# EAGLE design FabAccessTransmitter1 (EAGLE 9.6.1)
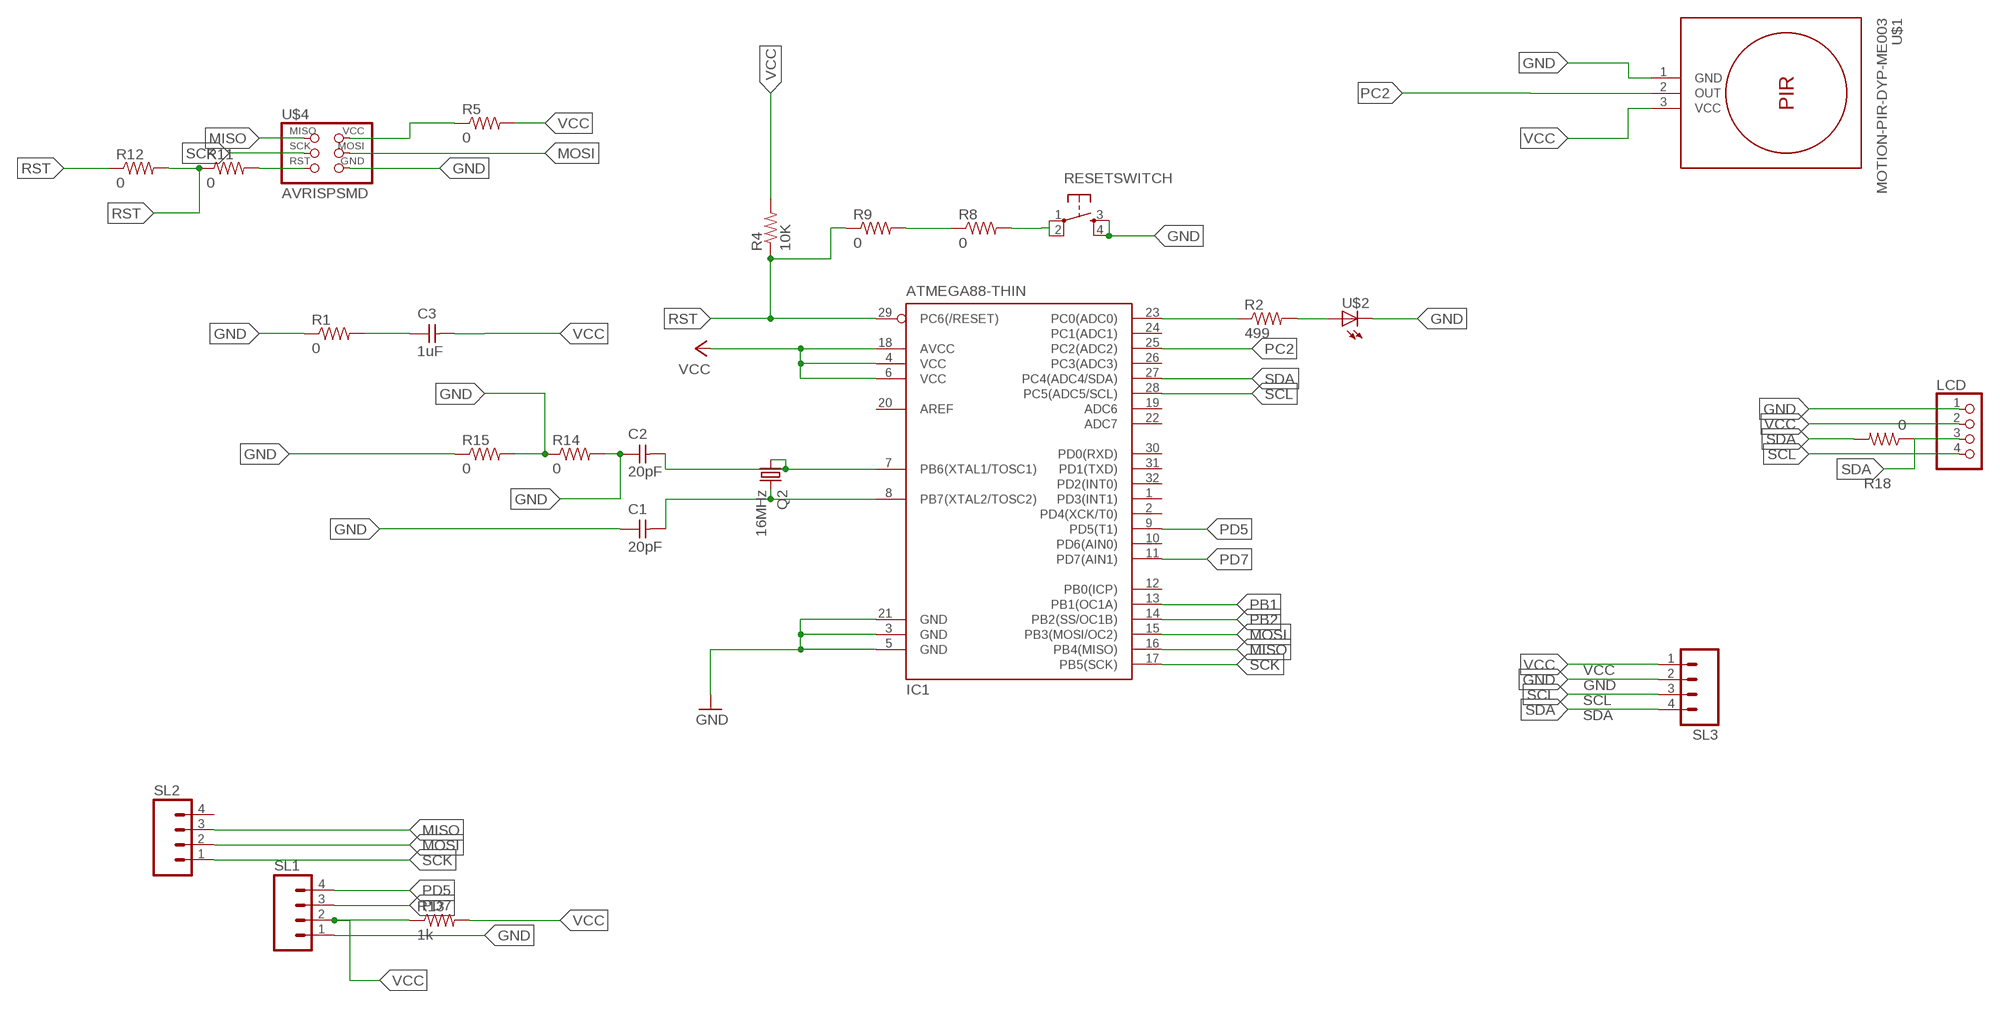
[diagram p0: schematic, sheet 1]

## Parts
C1  20pF  UNPOLARIZED_CAPACITOR1206  [1206]
C2  20pF  UNPOLARIZED_CAPACITOR1206  [1206]
C3  1uF  UNPOLARIZED_CAPACITOR1206  [1206]
IC1  ATMEGA88-THIN  [TQFP32-08THIN]
LCD  PINHD-1X4  [1X04]
Q2  16MHz  CSM-7X-DU  [CSM-7X-DU]
R1  0  RES-US1206  [R1206]
R2  499  RES-US1206  [R1206]
R4  10K  RESISTOR1206  [1206]
R5  0  RES-US1206  [R1206]
R8  0  RES-US1206  [R1206]
R9  0  RES-US1206  [R1206]
R11  0  RES-US1206  [R1206]
R12  0  RES-US1206  [R1206]
R13  1k  RES-US1206  [R1206]
R14  0  RES-US1206  [R1206]
R15  0  RES-US1206  [R1206]
R18  0  RESISTOR1206  [1206]
RESETSWITCH  6MM_SWITCH6MM_SWITCH  [6MM_SWITCH]
SL1  M04  [04P]
SL2  M04  [04P]
SL3  M04  [04P]
U$1  MOTION-PIR-DYP-ME003  [MOTION-PIR-DYP-ME003]
U$2  LED1206  [1206]
U$4  AVRISPSMD  [2X03SMD]

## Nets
GND: C1.1 C2.1 C3.1 IC1.3(GND) IC1.5(GND) IC1.21(GND) LCD.1 R1.1 R1.2 R14.1 R14.2 R15.1 R15.2 RESETSWITCH.3(S) RESETSWITCH.4(S1) SL1.1 SL3.2 U$1.1(GND) U$2.2(C) U$4.6(GND)
MISO: IC1.16(PB4(MISO)) SL2.3 U$4.1(MISO)
MOSI: IC1.15(PB3(MOSI/OC2)) SL2.2 U$4.4(MOSI)
N$1: IC1.23(PC0(ADC0)) R2.1
N$2: R2.2 U$2.1(A)
N$6: R8.1 R9.2
N$9: R8.2 RESETSWITCH.1(P) RESETSWITCH.2(P1)
PB1: IC1.13(PB1(OC1A))
PB2: IC1.14(PB2(SS/OC1B))
PC2: IC1.25(PC2(ADC2)) U$1.2(OUT)
PD5: IC1.9(PD5(T1)) SL1.4
PD7: IC1.11(PD7(AIN1)) SL1.3
RST: IC1.29(PC6(/RESET)) R4.1 R9.1 R11.1 R11.2 R12.1 R12.2 U$4.5(RST)
SCK: IC1.17(PB5(SCK)) SL2.1 U$4.3(SCK)
SCL: IC1.28(PC5(ADC5/SCL)) LCD.4 SL3.3
SDA: IC1.27(PC4(ADC4/SDA)) LCD.3 R18.1 R18.2 SL3.4
VCC: C3.2 IC1.4(VCC) IC1.6(VCC) IC1.18(AVCC) LCD.2 R4.2 R5.1 R5.2 R13.1 R13.2 SL1.2 SL3.1 U$1.3(VCC) U$4.2(VCC)
XTAL1: C2.2 IC1.7(PB6(XTAL1/TOSC1)) Q2.1
XTAL2: C1.2 IC1.8(PB7(XTAL2/TOSC2)) Q2.2
Unconnected: IC1.1(PD3(INT1)) IC1.2(PD4(XCK/T0)) IC1.10(PD6(AIN0)) IC1.12(PB0(ICP)) IC1.19(ADC6) IC1.20(AREF) IC1.22(ADC7) IC1.24(PC1(ADC1)) IC1.26(PC3(ADC3)) IC1.30(PD0(RXD)) IC1.31(PD1(TXD)) IC1.32(PD2(INT0)) SL2.4

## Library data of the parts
C1-C3 = FAB_Hello:UNPOLARIZED_CAPACITOR: unpolarized_capacitor
IC1 = fab:ATMEGA88-THIN
LCD = pinhead:PINHD-1X4: PIN HEADER
Q2 = FAB_Hello:CSM-7X-DU: SMD CRYSTAL; OC_FARNELL: unknown; OC_NEWARK: unknown
R1 R2 R5 R8 R9 R11-R15 = fab:RES-US: Resistor (US Symbol)
R4 R18 = FAB_Hello:RESISTOR
RESETSWITCH = FAB_Hello:6MM_SWITCH: OMRON SWITCH
SL1-SL3 = con-amp-quick:M04: AMP QUICK CONNECTOR; OC_FARNELL: unknown; OC_NEWARK: unknown
U$1 = diy-modules:MOTION-PIR-DYP-ME003: PIR Motion Sensor Module DYP-ME003 based on BISS0001 pyroelectic detector Click here to find device on ebay.com
U$2 = FAB_Hello:LED
U$4 = FAB_Hello:AVRISP

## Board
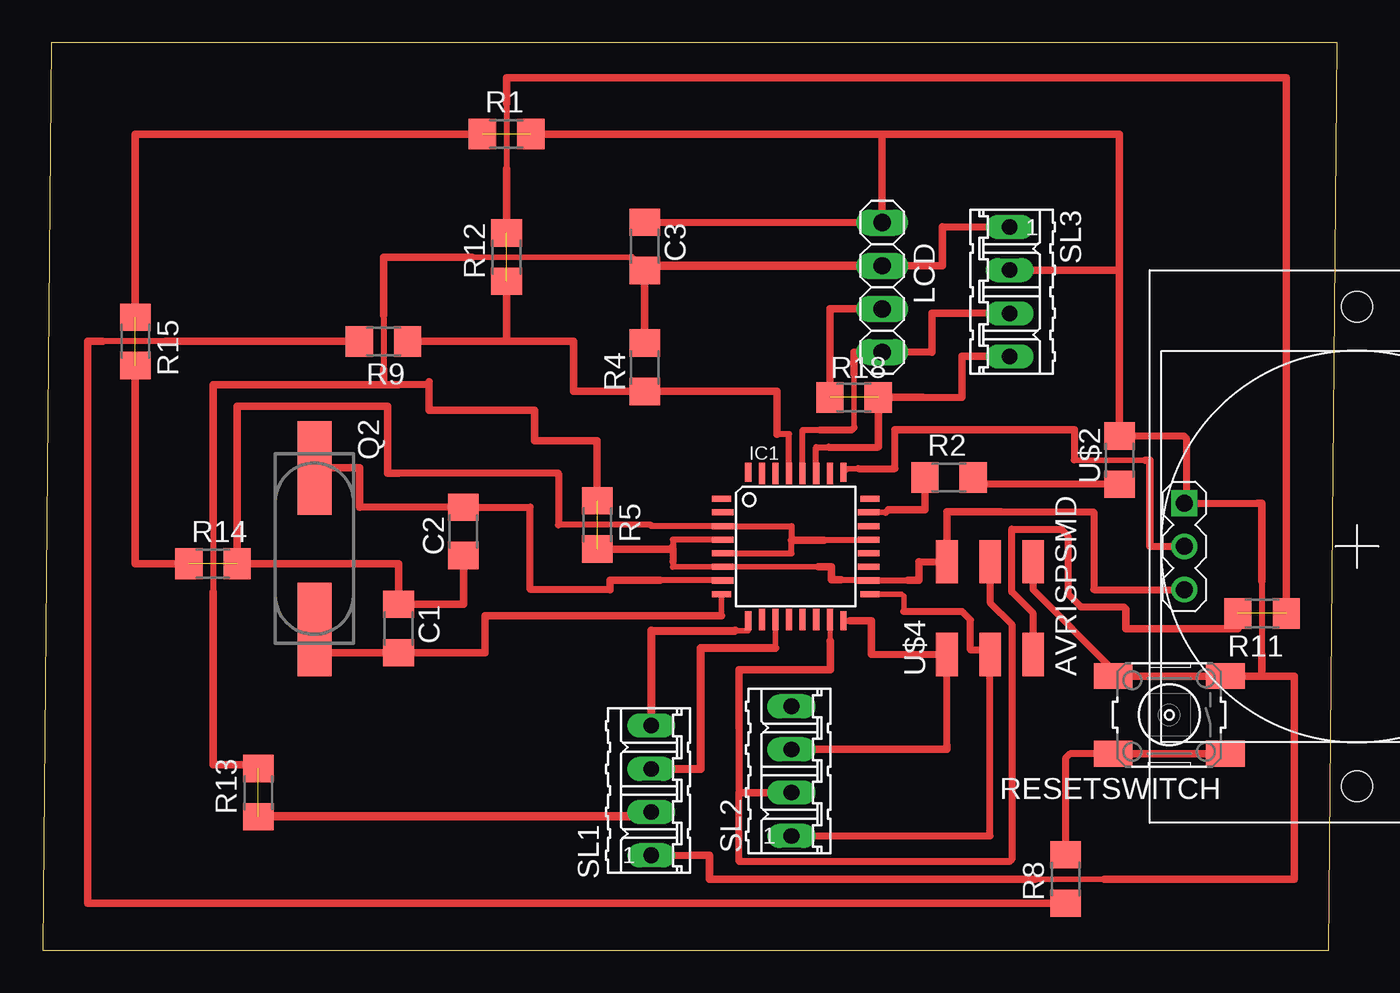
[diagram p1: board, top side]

Size 76.18 x 53.39 mm. Coordinates in mm from the lower left corner, seen from the top.
Outline: 0,0 75.67,0 76.18,53.39 0.51,53.39 0,0
Copper layers (1*16): Top 0.035mm / dielectric 1.5mm / Bottom 0.035mm
Design rules "default *": minimum track width 6mil, minimum drill 0.35mm, track to track 17mil, track to pad 17mil, pad to pad 17mil, via to via 17mil, smd to smd 17mil, copper to edge 40mil, drill to drill 6mil, minimum pad ring 10mil, minimum via ring 8mil, stop-mask expansion 4mil, vias tented up to drill 0mil, thermal gap 17mil

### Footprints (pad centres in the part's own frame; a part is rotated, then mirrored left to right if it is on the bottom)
1206 = smd 1.6 x 1.803: 1 -1.422,0; 2 1.422,0
TQFP32-08THIN = smd 1.118 x 0.356: 1 -4.369,2.8; 8 -4.369,-2.8; 17 4.369,-2.8; 24 4.369,2.8 | smd 1.27 x 0.356: 2 -4.293,2; 3 -4.293,1.2; 4 -4.293,0.4; 5 -4.293,-0.4; 6 -4.293,-1.2; 7 -4.293,-2; 18 4.293,-2; 19 4.293,-1.2; 20 4.293,-0.4; 21 4.293,0.4; 22 4.293,1.2; 23 4.293,2 | smd 0.356 x 1.118: 9 -2.8,-4.369; 16 2.8,-4.369; 25 2.8,4.369; 32 -2.8,4.369 | smd 0.356 x 1.27: 10 -2,-4.293; 14 1.2,-4.293; 15 2,-4.293; 26 2,4.293; 27 1.2,4.293; 31 -2,4.293 | smd 0.35 x 1.27: 11 -1.2,-4.293; 12 -0.4,-4.293; 13 0.4,-4.293; 28 0.4,4.293; 29 -0.4,4.293; 30 -1.2,4.293
1X04 = drill 1.016 long: 1 -3.81,0; 2 -1.27,0; 3 1.27,0; 4 3.81,0
CSM-7X-DU = smd 5.5 x 2: 1 -4.75,0; 2 4.75,0
R1206 = smd 1.6 x 1.803: 1 -1.422,0; 2 1.422,0
6MM_SWITCH = smd 2.286 x 1.524: 1 -3.302,2.286; 2 3.302,2.286; 3 -3.302,-2.286; 4 3.302,-2.286
04P = drill 0.914 long: 1 -3.81,0; 2 -1.27,0; 3 1.27,0; 4 3.81,0
MOTION-PIR-DYP-ME003 = drill 1 square: 1 -2.54,-10.16 | drill 1: 2 0,-10.16; 3 2.54,-10.16 | hole 1.8: -14.1,0; 14.1,0
2X03SMD = smd 2.54 x 1.27: 1 -2.54,2.54; 2 2.92,2.54; 3 -2.54,0; 4 2.92,0; 5 -2.54,-2.54; 6 2.92,-2.54

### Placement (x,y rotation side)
C1  20.96,18.92 270 top
C2  24.77,24.64 90 top
C3  35.43,41.4 270 top
IC1  44.32,23.75 0 top
LCD  49.4,38.99 270 top
Q2  16,23.62 270 top
R1  27.31,48.01 0 top
R2  53.34,27.81 0 top
R4  35.43,34.29 90 top
R5  32.64,25.02 270 top
R8  60.2,4.19 90 top
R9  20.07,35.81 180 top
R11  71.75,19.81 180 top
R12  27.31,40.77 90 top
R13  12.7,9.27 90 top
R14  10.03,22.73 0 top
R15  5.46,35.81 270 top
R18  47.75,32.51 0 top
RESETSWITCH  66.29,13.84 180 top
SL1  35.81,9.4 90 top
SL2  44.07,10.54 90 top
SL3  56.9,38.73 270 top
U$1  77.34,23.75 270 top
U$2  63.37,28.83 90 top
U$4  55.75,19.94 90 top

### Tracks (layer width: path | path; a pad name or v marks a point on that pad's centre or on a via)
GND  (3 unrouted)
  Top 0.33: 58.42,4.19 62.48,4.19 64.13,4.19 | IC1.21 48.62,24.13 47.75,24.13
  Top 0.356: 30.35,25.02 35.81,25.02 35.81,24.95 IC1.3 44.07,24.95 44.07,24.13 44.07,23.35 IC1.5 | 47.75,24.13 45.97,24.13 | 71.75,25.4 71.75,21.72 71.75,17.4
  Top 0.406: U$4.6 58.29,21.21 62.99,16.51 RESETSWITCH.4 64.01,16.13 | 67.31,26.29 71.5,26.29 | 67.31,26.29 U$1.1 | LCD.1 35.45,42.8 C3.1 | SL1.1 38.23,5.59 | 63.37,31.62 U$2.2 67.16,30.25 67.31,30.1 67.31,26.29 | 30.35,25.02 30.35,28.07 20.96,28.07 | R14.1 8.13,23.22
  Top 0.432: 71.75,17.4 71.75,16.13 | 45.97,24.13 44.07,24.13 | R14.1 5.46,22.73 R15.2 | C2.1 24.77,20.35 C1.1 20.96,22.73 R14.2 11.46,32 20.32,32 20.32,28.07 20.96,28.07 | R1.2 49.4,48.01 | 49.4,48.01 LCD.1 | 49.4,48.01 63.37,48.01 63.37,40 | 63.37,40 U$2.2 | SL3.2 63.37,40 | R1.1 5.46,48.01 R15.1 | 38.23,5.59 39.24,5.59 39.24,4.19 58.42,4.19 | 71.5,26.29 71.75,26.29 71.75,21.72 | RESETSWITCH.4 RESETSWITCH.3 71.75,16.13 | 62.48,4.19 73.66,4.19 73.66,16.13 71.75,16.13
MISO
  Top 0.356: IC1.16 47.5,19.38
  Top 0.406: 53.21,12.07 U$4.1 48.77,17.4
  Top 0.432: 47.5,19.38 48.77,19.38 48.77,17.4 | SL2.3 53.21,11.81 53.21,12.07
MOSI
  Top 0.305: IC1.15 46.32,18.16
  Top 0.406: U$4.4 55.75,20.45 57.02,19.18 57.02,5.33 56.9,5.21 40.99,5.21 40.99,9.27 40.99,13.08
  Top 0.432: 40.99,13.08 40.99,16.51 46.36,16.51 46.36,18.16 46.32,18.16 | SL2.2 40.99,9.27
N$1
  Top 0.33: 49.62,25.75 IC1.23
  Top 0.406: 49.62,25.75 49.78,25.91
  Top 0.432: 49.78,25.91 51.92,25.91 R2.1
N$2
  Top 0.406: R2.2 55.17,27.41 U$2.1
N$6
  Top 0.356: 7.24,35.81 3.56,35.81
  Top 0.432: R8.1 2.67,2.77 2.67,35.81 3.56,35.81 | R9.2 7.24,35.81
N$9
  Top 0.406: R8.2 60.2,11.3 60.45,11.56 RESETSWITCH.2
  Top 0.432: RESETSWITCH.2 RESETSWITCH.1
PC2
  Top 0.33: IC1.25 47.33,28.32 48.01,28.32 | 60.71,28.83 64.9,28.83
  Top 0.406: 48.01,28.32 50.16,28.32 50.16,30.61 | 65.15,23.75 U$1.2 | 60.71,30.61 60.71,28.83
  Top 0.432: 64.9,28.83 65.15,28.83 65.15,23.75 | 50.16,30.61 60.71,30.61
PD5
  Top 0.33: IC1.9 41.52,18.8 40.77,18.8
  Top 0.457: 35.81,18.8 40.77,18.8
  Top 0.483: 35.81,18.8 SL1.4
PD7
  Top 0.33: 43.12,17.78 IC1.11
  Top 0.483: SL1.3 38.73,10.67 38.73,17.78 43.12,17.78
RST  (2 unrouted)
  Top 0.356: IC1.29 43.92,30.35 43.2,30.35 | 27.31,49.78 27.31,45.97
  Top 0.406: 21.59,35.92 R9.1 | 58.74,16.95 U$4.5 58.29,19.81 57.02,21.08 57.02,24.77 59.94,24.77 60.33,24.38 60.33,20.96 61.09,20.19 63.63,20.19 63.75,20.07
  Top 0.432: R9.1 27.31,35.81 | 27.31,35.81 31.24,35.81 31.24,32.87 R4.1 43.2,32.87 43.2,30.35 | R12.1 27.31,35.81 | 27.31,45.97 R12.2 | 27.31,49.78 27.31,51.31 73.18,51.31 R11.1 | R11.2 70.33,18.92 63.75,18.92 63.75,20.07
SCK
  Top 0.33: IC1.17 50.55,20.95 50.67,20.83 50.67,19.94
  Top 0.406: 50.67,19.94 54.1,19.94 54.61,19.43 54.61,17.65 55.5,17.65 U$4.3 55.75,6.73 SL2.1
SCL
  Top 0.33: 47.75,30.73 47.75,33.91
  Top 0.356: IC1.28 44.72,30.61 45.72,30.61
  Top 0.406: 45.72,30.61 47.62,30.61 47.75,30.73 | 49.02,35.18 LCD.4 52.32,35.18 | SL3.3 54.61,37.47
  Top 0.432: 47.75,33.91 47.75,35.18 49.02,35.18 | 52.32,35.18 52.32,37.47 54.61,37.47
SDA  (1 unrouted)
  Top 0.356: IC1.27 45.52,29.59 46.25,29.59
  Top 0.406: 46.25,29.59 49.15,29.59 49.17,29.62 | 51.82,32.51 54.1,32.51
  Top 0.432: LCD.3 46.33,37.72 R18.1 | 51.82,32.51 R18.2 49.17,29.62 | 54.1,32.51 54.1,34.92 SL3.4
VCC  (2 unrouted)
  Top 0.33: 37.08,22.55 IC1.6 45.65,22.55 | 25.27,40.77 34.65,40.77 | 47.88,21.72 47.89,21.72 48.59,21.72 IC1.18
  Top 0.356: 10.03,25.02 10.03,21.08 | 20.07,37.34 20.07,34.16 | IC1.4 37.08,24.15 37.08,23.6 | 37.08,22.86 37.08,22.55 | 50.93,21.75 IC1.18 46.99,21.75 46.99,21.78
  Top 0.406: 51.56,22.86 U$4.2 | U$1.3 61.85,21.21 61.85,25.78 56.39,25.78 | R5.2 32.87,23.6 | 22.73,33.27 20.96,33.27 | 35.86,40.26 35.71,40.16 C3.2 34.65,40.77 | 52.96,42.55 SL3.1 | 37.08,22.86 37.08,23.6 37.08,23.77
  Top 0.432: 20.96,33.27 20.07,33.27 | 20.07,33.27 10.03,33.27 10.03,25.02 | 10.03,21.08 10.03,10.92 12.7,10.92 R13.2 | 22.73,33.43 22.73,33.27 22.73,31.75 28.96,31.75 28.96,29.97 32.64,29.97 R5.1 | R4.2 35.43,40.16 35.71,40.16 | 20.07,34.16 20.07,33.27 | 20.07,37.34 20.07,40.77 25.27,40.77 | R5.2 37.08,23.6 | 45.65,22.55 46.42,22.55 46.42,21.78 46.99,21.78 | 51.56,22.86 51.56,21.75 50.93,21.75 | LCD.2 52.96,40.26 52.96,42.55 | U$4.2 53.21,25.78 56.39,25.78 | SL1.2 35.81,7.87 | R13.1 12.7,7.87
  Top 0.508: LCD.2 35.86,40.26 | 35.81,7.87 12.7,7.87
XTAL1
  Top 0.356: IC1.7 36.32,21.75
  Top 0.406: 33.4,21.21 28.7,21.21 28.7,26.06 C2.2 18.67,26.06
  Top 0.432: Q2.1 18.67,28.37 18.67,26.06 | 33.4,21.21 33.4,21.75 36.32,21.75
XTAL2
  Top 0.33: 39.95,19.68 IC1.8
  Top 0.432: Q2.2 16,17.5 C1.2 26.04,17.5 26.04,19.68 39.95,19.68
